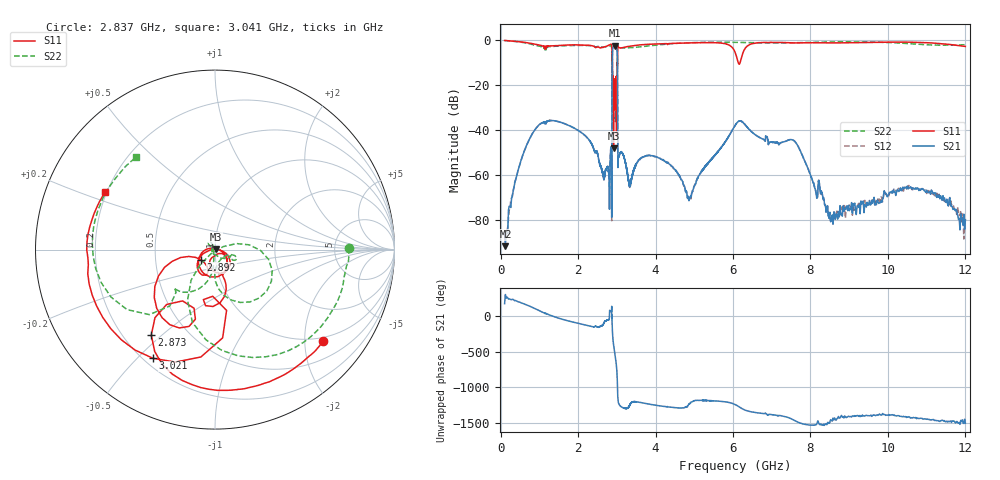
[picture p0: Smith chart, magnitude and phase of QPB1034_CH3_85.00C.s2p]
! TDS: k:\Engsetup\Winsaw\QPB1034_ALL
! Channel 1
! Ports=1 2
! seg 1=100.000000 1100.000000 51
! seg 2=1101.000000 1301.000000 201
! seg 3=1302.000000 2302.000000 101
! seg 4=2303.000000 3503.000000 1201
! seg 5=3504.000000 5204.000000 171
! seg 6=5205.000000 6405.000000 1201
! seg 7=6406.000000 8506.000000 211
! seg 8=8507.000000 12007.000000 176
! Points=3313
! FailCode=0
! Topology=ALL_SE(12)
!VNA Cal loaded =QPB1034_ALL_85C
!PS1(V)= 5.000
!PS(mA)= 0.439
!PS2(V)= 0.630
!PS(mA)= -0.004
!PS3(V)= 1.170
!PS(mA)= 0.000
!PS4(V)= 1.170
!PS(mA)= -0.001
!Temp (C)= 85.00
# MHz S DB R 50
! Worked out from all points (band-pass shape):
!   3313 points, 100 MHz to 12.01 GHz, reference 50 ohm
!   highest |S21| = -2.62 dB at 2.944 GHz (marker M1); lowest = -91.5 dB at 120 MHz (marker M2)
!   |S21| within 3 dB of the highest: 2.888 GHz to 3.01 GHz (122.7 MHz wide, 4.16 % of centre)
!   lowest |S11| = -48.2 dB at 2.915 GHz (marker M3), VSWR 1.01, Z = 50.3 + j0.238 ohm
!   |S11| at or under -10 dB: 2.887 GHz to 3.013 GHz (126.3 MHz wide, 4.28 % of centre); 3.014016 GHz to 3.016692 GHz (2.676 MHz wide, 0.0887 % of centre); 6.134 GHz to 6.189 GHz (55.06 MHz wide, 0.894 % of centre)
!   |S22| runs from -40.0 to -0.3 dB; largest |S21 - S12| = 0.0051
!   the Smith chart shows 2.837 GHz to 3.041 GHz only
!   S11 on the Smith chart (normalised r, x): 2.837 GHz: 0.90, -2.44; 2.873 GHz: 0.31, -0.46; 2.892 GHz: 0.85, -0.10; 3.021 GHz: 0.24, -0.56; 3.041 GHz: 0.19, +0.24
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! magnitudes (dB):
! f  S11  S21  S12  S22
! 100 MHz  -0.3  -85.7  -85.7  -0.3
! 120 MHz  -0.4  -91.5  -88.3  -0.4
! 240 MHz  -0.5  -73.8  -74.7  -0.6
! 500 MHz  -0.9  -55.0  -54.8  -1.0
! 1.1 GHz  -2.7  -36.5  -36.5  -3.2
! 2.434 GHz  -3.3  -49.7  -49.9  -3.2
! 2.802 GHz  -2.3  -63.5  -63.8  -2.7
! 2.837 GHz  -2.1  -49.4  -49.3  -2.6
! 2.873 GHz  -4.5  -32.3  -32.3  -13.3
! 2.892 GHz  -20.3  -4.3  -4.3  -19.6
! 2.915 GHz  -48.2  -2.9  -2.9  -20.1
! 2.944 GHz  -20.9  -2.6  -2.6  -25.4
! 3.002 GHz  -17.6  -4.1  -4.0  -31.3
! 3.021 GHz  -3.1  -28.5  -28.5  -3.6
! 3.041 GHz  -3.2  -52.1  -52.0  -3.4
! 4.874 GHz  -1.4  -70.0  -70.6  -1.3
! 5.406 GHz  -1.3  -53.7  -53.7  -1.1
! 6.2 GHz  -9.3  -36.0  -36.0  -1.2
! 7.596 GHz  -1.4  -45.0  -45.0  -1.3
! 8.507 GHz  -1.4  -79.4  -78.6  -1.0
! 10.65 GHz  -1.1  -65.7  -66.5  -1.9
! 12.01 GHz  -3.0  -79.8  -79.9  -2.2
